PROGRAM MAIN_CM

VAR CONSTANT
	
	cInitSpectrum 	: ST_CM_MagnitudeSpectrum_InitPars := (	nFFT_Length := cFFTLength, 
															nWindowLength := cWindowLength, 
															bTransformToDecibel:= FALSE, 
															eWindowType := E_CM_WindowType.eCM_HannWindow, 
															eScalingType := E_CM_ScalingType.eCM_RMS );
															
	cInitMC 		: ST_CM_MomentCoefficients_InitPars := ( nChannels := cFFTResult,
															 nOrder := E_CM_MCoefOrder.eCM_Mean,
															 bPopulationEstimates := TRUE );	
															 
	cInitBuffer			: ST_MA_MultiArray_InitPars := ( eTypeCode := eMA_TypeCode_LREAL, 
														 nDims := 1, 
														 aDimSizes := [cFFTResult]);															 

	cInitClassification	: ST_CM_DiscreteClassification_InitPars := (nChannels:= cFFTResult, 
																	nMaxClasses := cMaxClasses);
								
END_VAR

VAR	
	fbSpectrum			: FB_CMA_MagnitudeSpectrum :=(	stInitPars := cInitSpectrum, 
														nOwnID := eID_Spectrum, 
														aDestIDs := [eID_Sink, eID_MC],
														nResultBuffers   := 5 ); 
														
	fbMomCoeff			: FB_CMA_MomentCoefficients :=(	stInitPars := cInitMC, 
														nOwnID := eID_MC, 
														aDestIDs := [eID_BufferConverter, eID_SinkMC],
														nResultBuffers   := 5 ); 	

	fbBufferConverter	: FB_CMA_BufferConverting   :=( stInitPars := cInitBuffer,
														 nOwnID := eID_BufferConverter,
														 aDestIDs := [eID_Classify] ); 
																
														
	fbClassification	: FB_CMA_DiscreteClassification := (stInitPars := cInitClassification,
															nOwnID := eID_Classify, 
															aDestIDs := [eID_SinkClassify] );	
	
	// classification variables									
	aClassArgs			: ARRAY [1..cFFTResult, 1..cMaxClasses] OF LREAL;
	bConfigureClassifier: BOOL := TRUE;	
	nFreqBin            : UDINT;
	
	// Array for buffer converter: only copy second column (averaged spectrum)
	aStartIdx 			: ARRAY[1..2] OF UDINT := [0,1];
	
	fbErrHist			: FB_HRErrHist; // error monitoring
END_VAR

// call cofiguration of classifier: here onyl in first cycle
MAIN_CM.ConfigClassification();

// calculate spectrum
MAIN_CM.SpectrumCall();

// average result of spectrum call
MAIN_CM.AverageCall();

// do classification
MAIN_CM.ExecuteClassification();

ACTION AverageCall:


// Average 
fbMomCoeff.CallEx(nAppendData := cNumAverage, bResetData := TRUE);
IF fbMomCoeff.bError THEN
	fbErrHist.AddError(bErr:=TRUE, hrErrCode:=fbMomCoeff.hrErrorCode, sErrSource:='MAIN_CM.fbMomCoeff'); // error monitoring
	// ToDo: if error
END_IF
END_ACTION

ACTION ConfigClassification:
(*--------- Configure classifier args ---------*)
IF bConfigureClassifier THEN
	// 
	FOR nFreqBin := 1 TO cFFTResult DO			
		// Classification configuration
		
		aClassArgs[nFreqBin, 1] := cThresholdBroadband;

		// set another threshold for window of approx 36 Hz to 61 Hz	
		IF nFreqBin > 30 THEN  // 30*fs/N = 36.621
			IF nFreqBin < 50 THEN  // 50*fs/N = 61.035
				aClassArgs[nFreqBin, 1] := cThreshold50Hz;	
			END_IF			
		END_IF			
	END_FOR		
	// call configure method
	fbClassification.Configure(pArg := ADR(aClassArgs), nArgSize := SIZEOF(aClassArgs));
	IF NOT fbClassification.bError THEN
		// reset for next configuration
		bConfigureClassifier := FALSE;
	ELSE
		fbErrHist.AddError(bErr := TRUE, hrErrCode := fbClassification.hrErrorCode, sErrSource := 'MAIN_CM.fbClassification.Configure');
	END_IF								
END_IF
END_ACTION

ACTION ExecuteClassification:

// (1) perform buffer conversion to only pass averaged spectrum to classifier 
// (2) execute classification

// (1)
fbBufferConverter.Copy1D(nWorkDimIn := 0, 
						 nWorkDimOut := 0,
						 nElements := 0,
						 pStartIndexIn 	:= ADR(aStartIdx),
						 pStartIndexOut := 0,
						 nOptionPars := 0);
IF fbBufferConverter.bError THEN
	fbErrHist.AddError(bErr := TRUE, hrErrCode := fbBufferConverter.hrErrorCode, sErrSource := 'MAIN_CM.fbBufferConverter');
END_IF

// (2) 
fbClassification.Call(bError => , hrErrorCode => );
IF fbClassification.bError THEN
	fbErrHist.AddError(bErr := TRUE, hrErrCode := fbClassification.hrErrorCode, sErrSource := 'MAIN_CM.fbClassification.Call');
END_IF
END_ACTION

ACTION SpectrumCall:


// Call spectrum 
fbSpectrum.Call();
IF fbSpectrum.bError THEN
	fbErrHist.AddError(bErr:=TRUE, hrErrCode:=fbSpectrum.hrErrorCode, sErrSource:='MAIN_CM.fbSpectrum'); // error monitoring
	// ToDo: if error
END_IF
END_ACTION

END_PROGRAM
